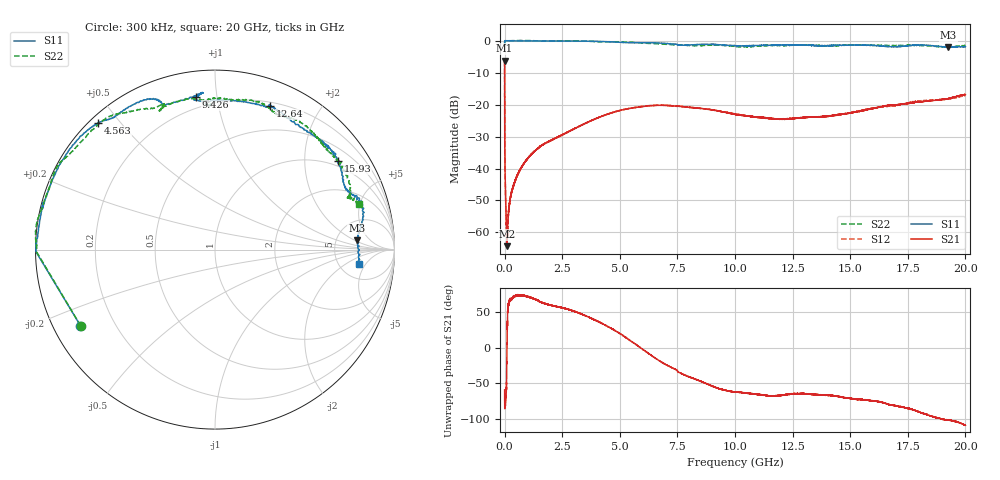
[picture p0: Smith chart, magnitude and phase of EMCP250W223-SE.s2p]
!EMCP250W223
!Johanson Technology Inc.
!www.johansontechnology.com
!Test Board Conditions:
!Substrate Type  RO4350B
!Substrate Thickness  10 mil
!Substrate Dk  3.66
!TL Type: GCPW
!TL Trace Width  20 mil
!TL Gap  10 mil
!PART MODE SINGLE ENDED (AKA BYPASS)
!DUT TOPOLOGY	SERIES-SHUNT
# MHz S  dB  R 50
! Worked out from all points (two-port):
!   20001 points, 300 kHz to 20 GHz, reference 50 ohm
!   highest |S21| = -6.23 dB at 300 kHz (marker M1); lowest = -64.3 dB at 104.3 MHz (marker M2)
!   |S21| within 3 dB of the highest: start of sweep to 563 kHz
!   lowest |S11| = -2.0 dB at 19.27 GHz (marker M3), VSWR 8.59, Z = 399 + j110 ohm
!   |S11| at or under -10 dB: nowhere
!   |S22| runs from -2.0 to 0.1 dB; largest |S21 - S12| = 0.0072
!   S11 on the Smith chart (normalised r, x): 300 kHz: 0.08, -0.26; 4.563 GHz: 0.02, +0.44; 9.426 GHz: 0.14, +0.87; 12.64 GHz: 0.24, +1.43; 15.93 GHz: 0.83, +2.89; 20 GHz: 7.71, -3.49
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0.3  -1.30 -150.6  -6.23 -59.4  -6.21 -59.7  -1.30 -150.4
104.298  -0.04 178.9  -64.29 5.7  -62.81 9.4  -0.06 179.3
162.298  -0.02 178.1  -54.88 58.8  -54.86 60.7  -0.06 178.6
294.296  -0.04 176.8  -47.66 68.9  -47.74 68.4  -0.03 177.6
508.292  -0.09 174.2  -42.97 72.9  -42.90 72.8  0.02 176.0
1056.284  -0.09 168.6  -36.42 71.3  -36.41 71.8  0.02 170.5
2144.268  -0.14 162.3  -30.75 58.6  -30.70 58.5  -0.10 157.1
3334.25  -0.14 146.1  -26.44 47.4  -26.48 47.2  -0.11 150.1
4563.232  -0.35 132.6  -22.77 28.3  -22.76 28.1  -0.40 139.1
6667.2  -0.72 114.3  -20.25 -17.4  -20.19 -17.8  -1.01 119.3
7600.186  -1.40 107.6  -20.55 -35.4  -20.57 -35.1  -1.32 109.4
8504.172  -1.17 95.3  -21.22 -47.2  -21.20 -47.6  -1.57 111.2
9426.159  -1.35 97.1  -22.20 -58.9  -22.20 -58.0  -1.46 97.6
10000.15  -1.57 96.3  -23.06 -62.3  -22.89 -62.1  -1.77 91.7
11343.13  -1.48 71.5  -24.14 -67.1  -24.30 -67.1  -1.51 91.8
12644.11  -1.34 68.9  -24.27 -64.8  -24.19 -65.1  -1.40 78.5
13334.1  -1.51 63.0  -23.87 -65.5  -23.86 -66.0  -1.42 70.5
15933.06  -1.45 35.7  -21.30 -74.8  -21.23 -76.0  -1.45 47.7
16667.05  -1.86 27.5  -20.25 -80.0  -20.52 -79.8  -1.54 44.5
18028.03  -1.42 16.0  -19.13 -90.9  -18.98 -90.9  -1.50 29.3
19266.01  -2.03 3.7  -18.16 -101.9  -18.29 -103.2  -2.03 21.3
20000  -1.87 -5.6  -16.86 -109.4  -17.08 -107.3  -1.48 17.5
